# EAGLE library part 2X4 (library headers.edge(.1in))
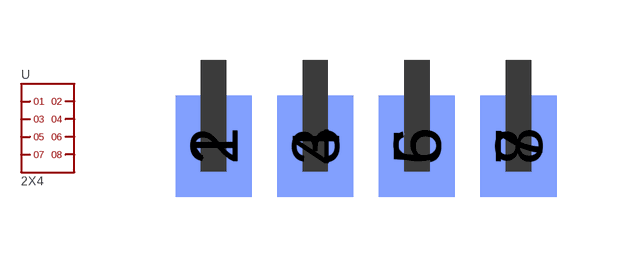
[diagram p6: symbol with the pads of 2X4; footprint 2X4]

Designator prefix -

## 2X4  [2X4]
1  1
2  2
3  3
4  4
5  5
6  6
7  7
8  8

## Footprint 2X4 (pad centres in mm)
smd 1.905 x 2.54: 1 0,-2.159; 3 2.54,-2.159; 5 5.08,-2.159; 7 7.62,-2.159
smd 1.905 x 2.54 bottom: 2 0,-2.159; 4 2.54,-2.159; 6 5.08,-2.159; 8 7.62,-2.159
